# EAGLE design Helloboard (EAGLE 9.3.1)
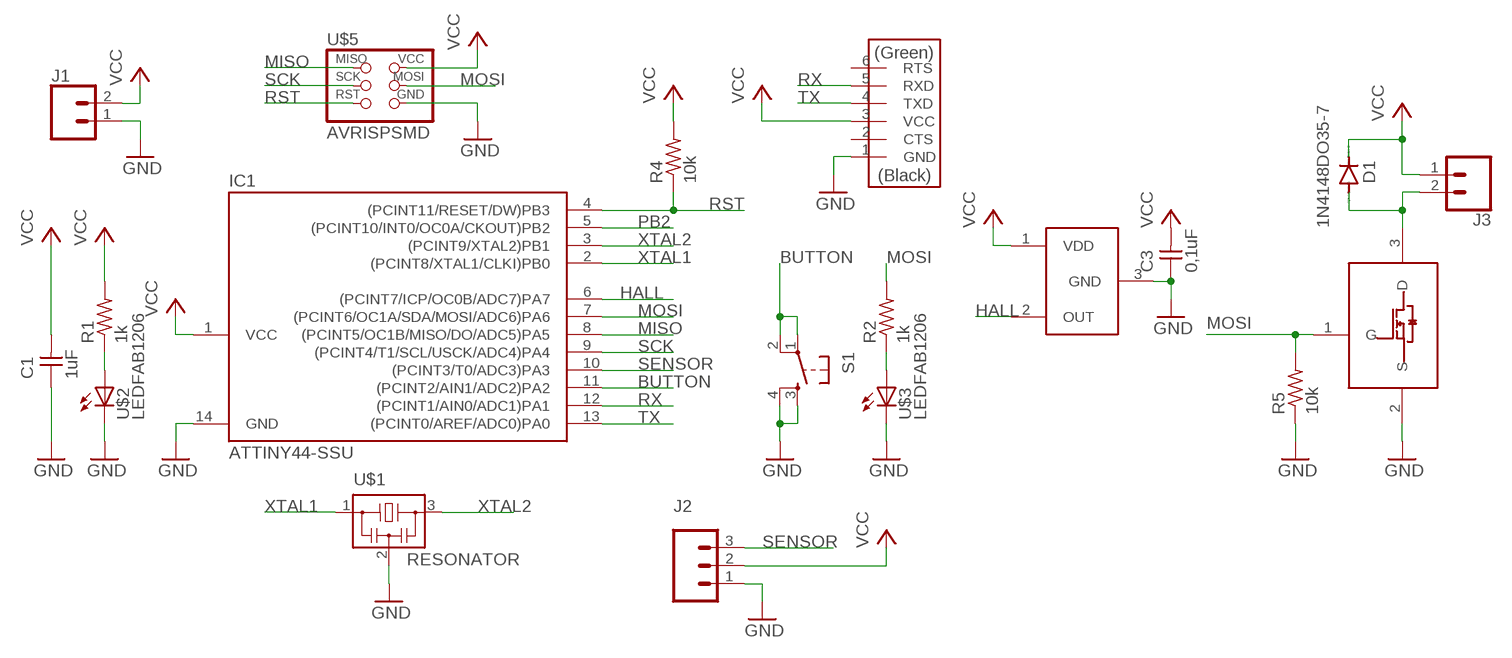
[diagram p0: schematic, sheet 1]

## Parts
C1  1uF  CAP-UNPOLARIZED  [C1206]
C3  0,1uF  CAP-UNPOLARIZED  [C1206]
D1  1N4148DO35-7  [DO35-7]
IC1  ATTINY44-SSU  [SOIC14]
J1  CONN_02POLAR  [MOLEX-1X2]
J2  CONN_03POLAR  [MOLEX-1X3]
J3  CONN_02POLAR  [MOLEX-1X2]
R1  1k  RES-US1206FAB  [R1206FAB]
R2  1k  RES-US1206FAB  [R1206FAB]
R4  10k  RES-US1206FAB  [R1206FAB]
R5  10k  RES-US1206FAB  [R1206FAB]
S1  6MM_SWITCH6MM_SWITCH  [6MM_SWITCH]
U1  HALL-SWITCH-S5712  [SOT23]
U$1  RESONATOR  [EFOBM]
U$2  LEDFAB1206  [LED1206FAB]
U$3  LEDFAB1206  [LED1206FAB]
U$5  AVRISPSMD  [2X03SMD]
U$6  FTDI-SMD-HEADER  [1X06SMD]
U$7  FET-1A-30V-PMF250XNESOT23  [SOT23]

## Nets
BUTTON: IC1.11((PCINT2/AIN1/ADC2)PA2) S1.1(P) S1.2(P1)
GND: C1.1 C3.1 IC1.14(GND) J1.1 J2.1 R5.1 S1.3(S) S1.4(S1) U1.3(GND) U$1.2 U$2.2(C) U$3.2(C) U$5.6(GND) U$6.1(GND) U$7.2(S)
HALL: IC1.6((PCINT7/ICP/OC0B/ADC7)PA7) U1.2(OUT)
MISO: IC1.8((PCINT5/OC1B/MISO/DO/ADC5)PA5) U$5.1(MISO)
MOSI: IC1.7((PCINT6/OC1A/SDA/MOSI/ADC6)PA6) R2.2 R5.2 U$5.4(MOSI) U$7.1(G)
N$1: R1.1 U$2.1(A)
N$2: D1.A J3.2 U$7.3(D)
N$3: R2.1 U$3.1(A)
PB2: IC1.5((PCINT10/INT0/OC0A/CKOUT)PB2)
RST: IC1.4((PCINT11/RESET/DW)PB3) R4.1 U$5.5(RST)
RX: IC1.12((PCINT1/AIN0/ADC1)PA1) U$6.5(RXD)
SCK: IC1.9((PCINT4/T1/SCL/USCK/ADC4)PA4) U$5.3(SCK)
SENSOR: IC1.10((PCINT3/T0/ADC3)PA3) J2.3
TX: IC1.13((PCINT0/AREF/ADC0)PA0) U$6.4(TXD)
VCC: C1.2 C3.2 D1.C IC1.1(VCC) J1.2 J2.2 J3.1 R1.2 R4.2 U1.1(VDD) U$5.2(VCC) U$6.3(VCC)
XTAL1: IC1.2((PCINT8/XTAL1/CLKI)PB0) U$1.1
XTAL2: IC1.3((PCINT9/XTAL2)PB1) U$1.3
Unconnected: U$6.2(CTS) U$6.6(RTS)

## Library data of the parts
C1 C3 = fab:CAP-UNPOLARIZED
D1 = diode:1N4148: DIODE
IC1 = fab:ATTINY44
J1 J3 = OPENBOT:CONN_02: Multi connection point. Often used as Generic Header-pin footprint for 0.1 inch spaced/style header connections; SF_ID: PRT-09918
J2 = OPENBOT:CONN_03: Multi connection point. Often used as Generic Header-pin footprint for 0.1 inch spaced/style header connections On any of the 0.1 inch spaced packages, you can populate with these: Break Away Headers - Straight (PRT-00116) Break Away Male Headers - Right Angle (PRT-00553) Female Headers (PRT-00115)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; PROD_ID: CONN-08625; SF_ID: PRT-08096
R1 R2 R4 R5 = fab:RES-US: Resistor (US Symbol)
S1 = fab:6MM_SWITCH: OMRON SWITCH
U1 = sensor:HALL-SWITCH-S5712
U$1 = fab:RESONATOR
U$2 U$3 = fab:LED: LED
U$5 = fab:AVRISP
U$6 = fab:FTDI-SMD-HEADER
U$7 = power:FET-1A-30V-PMF250XNE

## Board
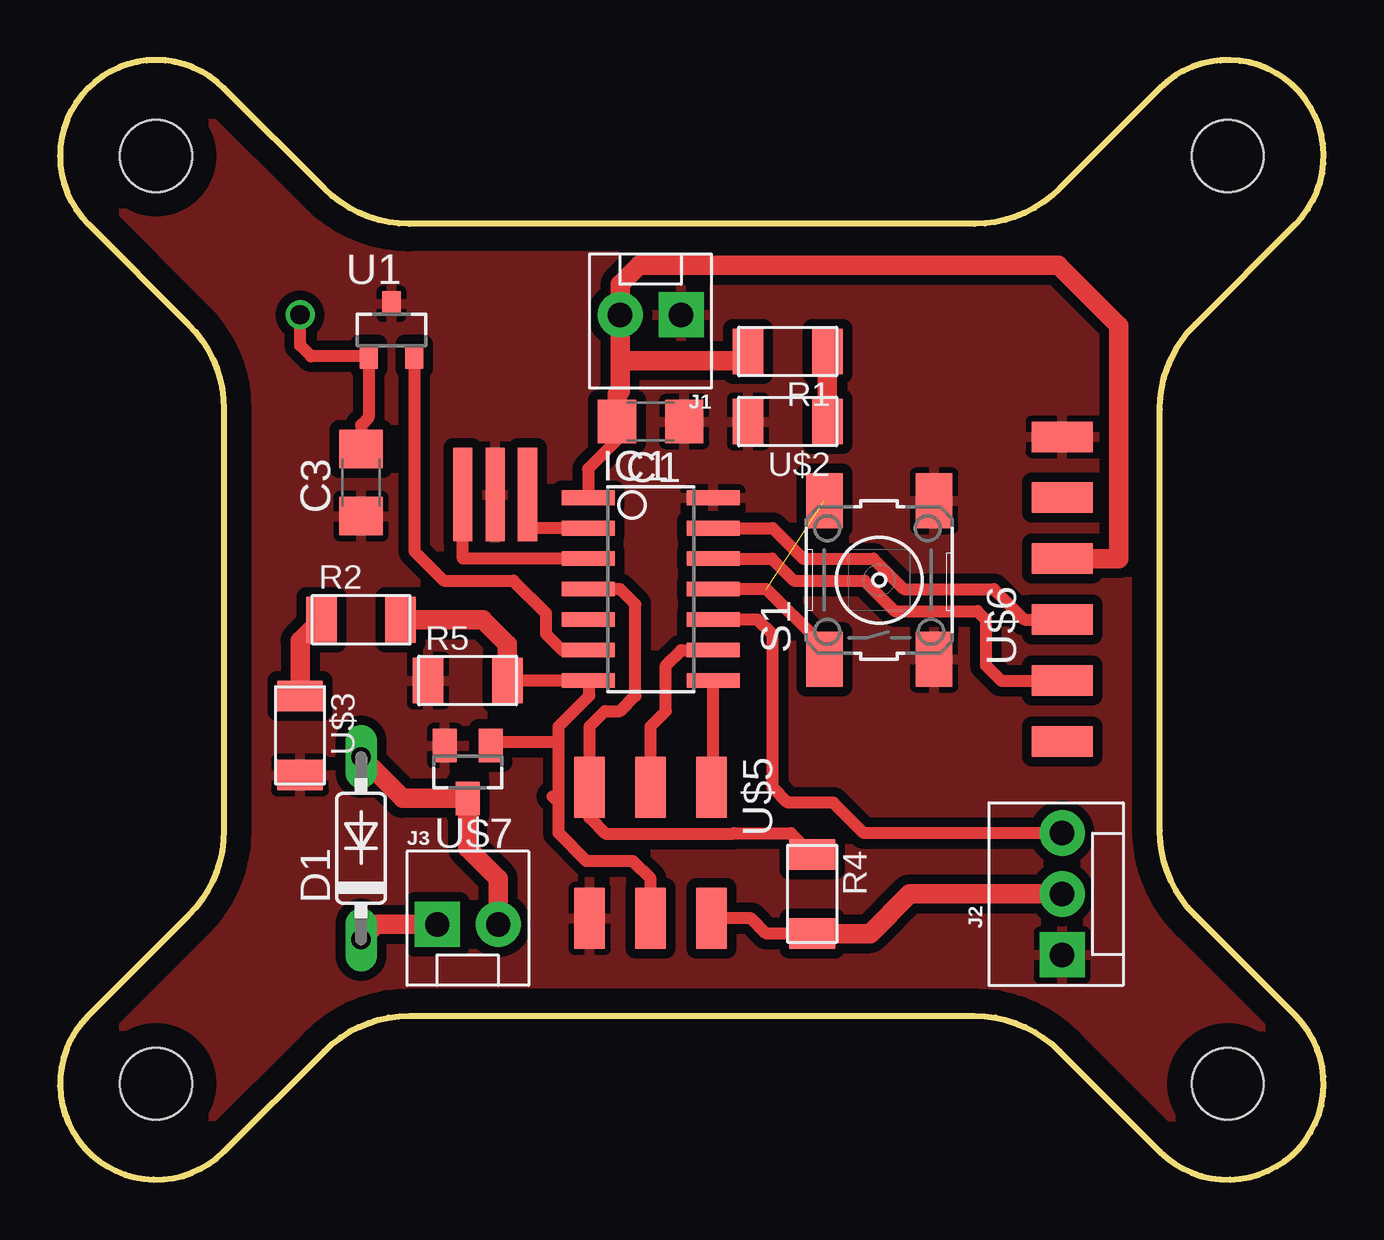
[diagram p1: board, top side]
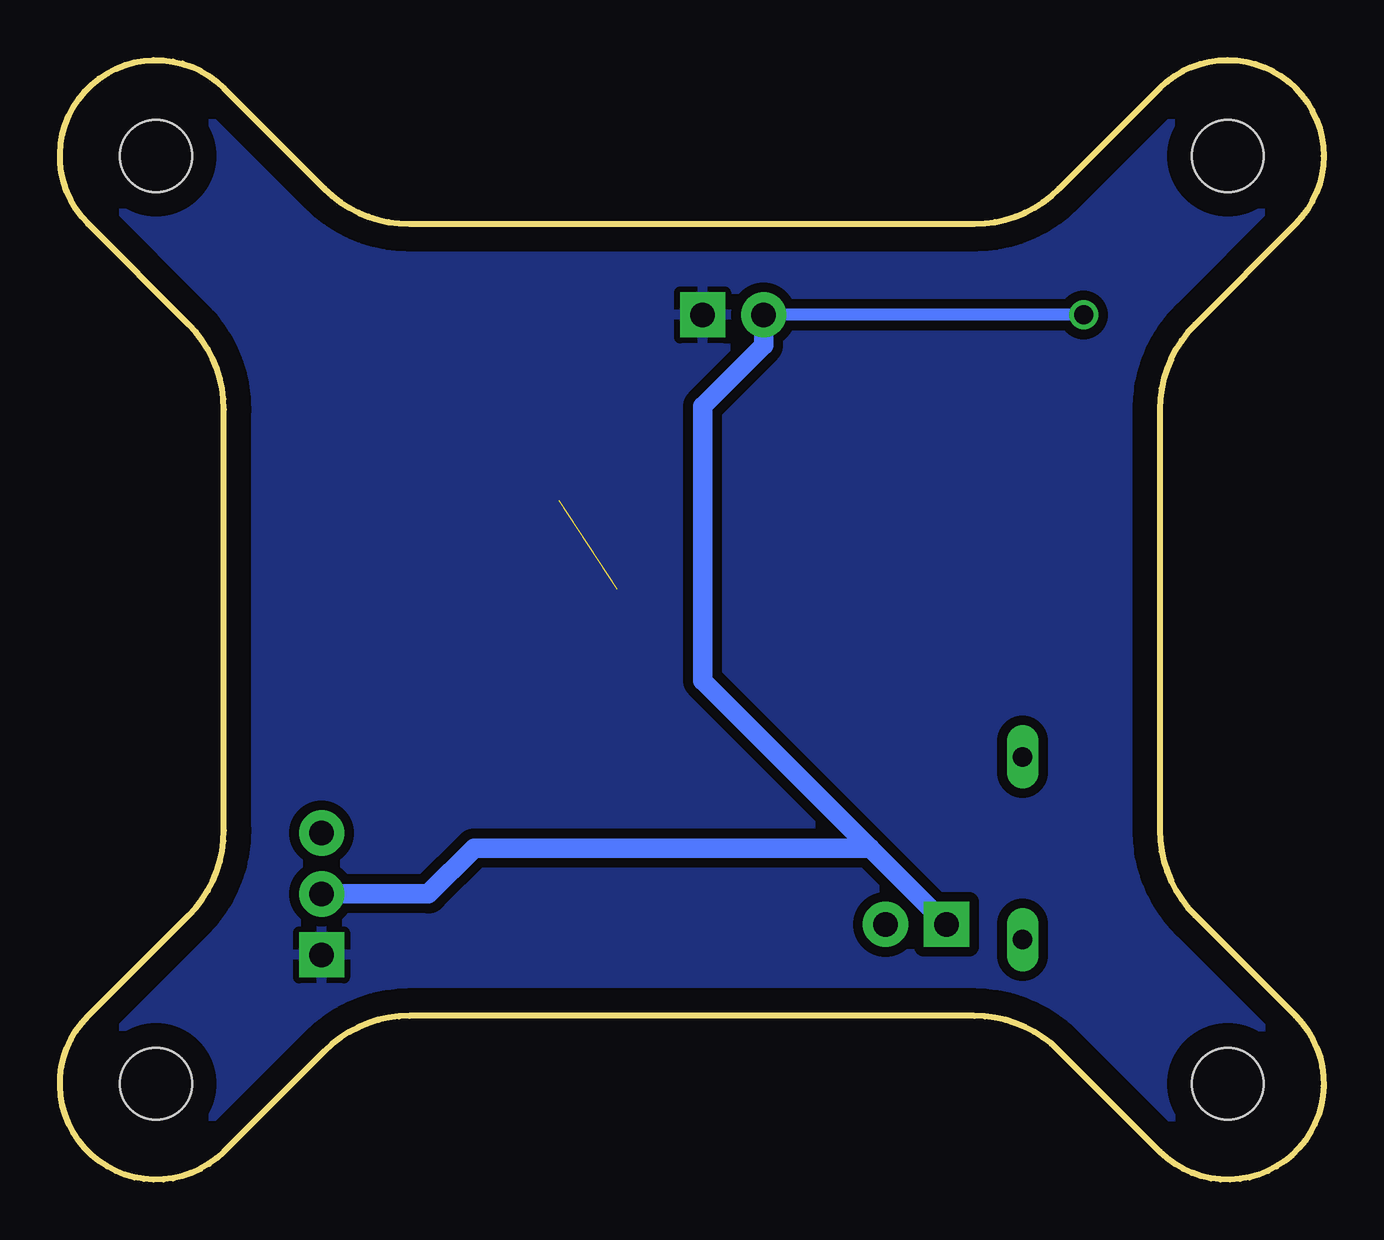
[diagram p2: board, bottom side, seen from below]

Size 52.66 x 46.66 mm. Coordinates in mm from the lower left corner, seen from the top.
Outline: 11.02,41.29 6.83,45.48 arc180 1.17,39.83 5.36,35.64 arc-45 6.83,32.1 6.83,14.56 arc-45 5.36,11.02 1.17,6.83 arc180 6.83,1.17 11.02,5.36 arc-45 14.56,6.83 38.1,6.83 arc-45 41.64,5.36 45.83,1.17 arc180 51.49,6.83 47.29,11.02 arc-45 45.83,14.56 45.83,32.1 arc-45 47.29,35.64 51.49,39.83 arc180 45.83,45.48 41.64,41.29 arc-45 38.1,39.83 14.56,39.83 arc-45 11.02,41.29
Copper layers (1*16): Top 0.035mm / dielectric 1.5mm / Bottom 0.035mm
Design rules "default *": minimum track width 15mil, minimum drill 0.35mm, track to track 16mil, track to pad 16mil, pad to pad 16mil, via to via 16mil, smd to smd 6mil, copper to edge 40mil, drill to drill 6mil, minimum pad ring 10mil, minimum via ring 8mil, stop-mask expansion 4mil, vias tented up to drill 0mil, thermal gap 10mil
Holes 3 mm at 4,42.66 48.66,42.66 4,4 48.66,4

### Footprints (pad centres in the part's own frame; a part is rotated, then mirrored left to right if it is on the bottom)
C1206 = smd 1.6 x 1.8: 1 -1.4,0; 2 1.4,0
DO35-7 = drill 0.813 long: A 3.81,0; C -3.81,0
SOIC14 = smd 0.61 x 2.21: 1 -3.81,-2.603; 2 -2.54,-2.603; 3 -1.27,-2.603; 4 0,-2.603; 5 1.27,-2.603; 6 2.54,-2.603; 7 3.81,-2.603; 8 3.81,2.603; 9 2.54,2.603; 10 1.27,2.603; 11 0,2.603; 12 -1.27,2.603; 13 -2.54,2.603; 14 -3.81,2.603
MOLEX-1X2 = drill 1.016 pad 1.88 square: 1 0,0 | drill 1.016 pad 1.88: 2 2.54,0
MOLEX-1X3 = drill 1.016 pad 1.88 square: 1 0,0 | drill 1.016 pad 1.88: 2 2.54,0; 3 5.08,0
R1206FAB = smd 1.27 x 1.905: 1 -1.651,0; 2 1.651,0
6MM_SWITCH = smd 2.286 x 1.524: 1 -3.302,2.286; 2 3.302,2.286; 3 -3.302,-2.286; 4 3.302,-2.286
SOT23 = smd 0.762 x 1.016: 1 -0.95,-1.1; 2 0.95,-1.1; 3 0,1.1
EFOBM = smd 0.8 x 3.9: 1 -1.35,0; 2 0,0; 3 1.35,0
LED1206FAB = smd 1.27 x 1.905: 1 -1.651,0; 2 1.651,0
2X03SMD = smd 2.54 x 1.27: 1 -2.54,2.54; 2 2.92,2.54; 3 -2.54,0; 4 2.92,0; 5 -2.54,-2.54; 6 2.92,-2.54
1X06SMD = smd 2.54 x 1.27: 1 0,6.35; 2 0,3.81; 3 0,1.27; 4 0,-1.27; 5 0,-3.81; 6 0,-6.35
SOT23' = smd 1 x 1.4: 1 -0.95,-1.1; 2 0.95,-1.1; 3 0,1.1

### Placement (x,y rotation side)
C1  24.61,31.59 180 top
C3  12.54,29.05 90 top
D1  12.54,13.81 90 top
IC1  24.61,24.61 270 top
J1  25.88,36.04 180 top
J2  41.75,9.37 90 top
J3  15.72,10.64 0 top
R1  30.32,34.51 180 top
R2  12.54,23.34 0 top
R4  31.34,11.91 270 top
R5  16.99,20.8 0 top
S1  34.13,24.99 90 top
U1  13.81,35.4 0 top
U$1  18.13,28.54 180 top
U$2  30.32,31.59 180 top
U$3  10,18.51 270 top
U$5  24.61,13.81 270 top
U$6  41.75,24.61 0 top
U$7  FET-1A-30V-PMF250XNESOT23  [SOT23']  16.99,16.99 180 top

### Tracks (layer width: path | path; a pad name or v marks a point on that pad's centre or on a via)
BUTTON  (1 unrouted)
  Top 0.508: S1.1 31.59,21.94 31.59,22.45 29.43,24.61 IC1.11
GND
  pour Top: -5.87,53.18 56.99,53.18 56.99,-3.33 -5.87,-3.33
  pour Bottom: -3.33,50.64 54.45,50.64 54.45,-0.79 -3.33,-0.79
HALL
  Top 0.508: U1.2 14.76,26.2 16,24.96 18.89,24.96 20.24,23.62 20.24,22.76 20.93,22.07 IC1.6
MISO
  Top 0.508: U$5.1 27.21,16.42 IC1.8
MOSI
  Top 0.508: U$5.4 24.61,12.54 23.87,13.28 21.94,13.28 20.77,14.45 20.77,15.72 | 20.77,15.72 20.77,18.26 | 20.77,18.26 20.77,18.89 22.06,20.17 22.06,20.75 IC1.7 R5.2 | 20.52,15.97 20.77,15.72 | U$7.1 18.11,18.26 20.77,18.26
  Top 0.813: R2.2 17.62,23.34 18.64,22.32 R5.2
N$1
  Top 0.813: R1.1 U$2.1
N$2
  Top 0.813: J3.2 18.26,12.54 16.99,13.81 U$7.3 14.28,15.89 D1.A
N$3
  Top 0.813: R2.1 10,22.45 U$3.1
RST
  Top 0.508: IC1.4 23.34,24.61 23.97,23.97 23.97,20.16 23.34,19.53 22.7,19.53 22.07,18.89 U$5.5 22.07,15.08 22.73,14.42 28.06,14.42 28.08,14.45 30.45,14.45 R4.1
RX
  Top 0.508: IC1.12 29.67,25.88 30.58,24.96 33.52,24.96 34.79,23.69 38.22,23.69 38.58,23.34 38.58,21.43 39.21,20.8 U$6.5
SCK
  Top 0.508: IC1.9 25.88,22.07 25.24,21.43 25.24,19.53 24.61,18.89 U$5.3
SENSOR
  Top 0.508: IC1.10 29.05,23.34 29.69,22.7 29.69,16.35 30.32,15.72 32.23,15.72 33.5,14.45 J2.3
TX
  Top 0.508: IC1.13 29.69,27.15 30.96,25.88 33.89,25.88 35.16,24.61 38.91,24.61 40.18,23.34 U$6.4
VCC  (via drill 0.8)
  Top 0.508: C1.2 23.21,30.83 22.01,29.62 IC1.1 | R4.2 29.43,10.26 28.8,10.89 U$5.2 | C3.2 12.54,31.46 12.56,31.46 12.86,31.76 U1.1 10.47,34.3 10,34.77 v10,36.04
  Top 0.813: U$5.2 | C1.2 23.21,32.73 23.34,32.86 23.34,34.13 | R4.2 33.75,10.26 35.4,11.91 J2.2 | D1.C 13.18,10.64 J3.1 | 23.34,34.13 J1.2 23.34,37.31 24.13,38.1 41.6,38.1 44.12,35.57 44.12,25.88 U$6.3 41.12,25.88 | R1.2 28.29,34.13 23.34,34.13
  Bottom 0.508: v10,36.04 J1.2
  Bottom 0.813: J3.1 18.89,13.81 | 18.89,13.81 35.4,13.81 37.31,11.91 J2.2 | 18.89,13.81 25.88,20.8 25.88,32.23 23.34,34.77 J1.2
XTAL1
  Top 0.508: IC1.2 19.48,27.15 U$1.1
XTAL2
  Top 0.508: IC1.3 16.78,25.88 U$1.3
